| TEXAS INSTRUMENTS INCORPORATED
| Standard Linear and Logic Group
| IBIS Model of SN74LVC240A
| OCTAL BUFFER/DRIVER WITH 3-STATE OUTPUTS
| This file contains package information for the following:
|  SSOP 20-pin (DB) package as [Component] LVC240A_DB
|  TVSOP 20-pin (DGV) package as [Component] LVC240A_DGV
|  SOIC 20-pin (DW) package as [Component] LVC240A_DW
|  SOP 20-pin (NS) package as [Component] LVC240A_NS
|  TSSOP 20-pin (PW) package as [Component] LVC240A_PW
| This device can be powered at the following Vccs:
|  1.8 volt Vcc
|  2.5 volt Vcc
|  2.7 volt Vcc
|  3.3 volt Vcc
| This file provides unique models under the [Model Selector] for each Vcc.
| For operation at a specific Vcc, select the appropriate model after each
| [Model Selector] keyword.
[IBIS Ver]   3.2
[Comment char]  |_char
[File Name]   sn74lvc240a.ibs
[File Rev]   1.1 | e_die
[Date]   March 10, 2003
[Source]   Data created from TI-SPICE simulations at TI-SLL.
[Notes]   The following is an IBIS list for the LVC240A.
   Please contact sllibis@ti.com with questions and
   comments concerning SLL IBIS models.
   This IBIS model is created from a BA (back annotated
   netlist).
   - Power-clamp data has been deleted since there is no
   power-clamp diode in the device.
   - Due to the fact that the device is 5-V input
   tolerant, the pullup data has some non-monotonic warnings.
[Disclaimer] Property of Texas Instruments Incorporated.  Unauthorized
   reproduction and/or distribution is strictly prohibited.
   This product is protected under copyright law.
   Created  2003, (C) Copyright  2003, Texas Instruments
   Incorporated, All Rights Reserved
   UNLESS THERE IS A SIGNED, WRITTEN AGREEMENT TO THE
   CONTRARY, TEXAS INSTRUMENTS (TI) IS PROVIDING THE IBIS
   MODELS  AND WITHOUT ANY WARRANTY, EXPRESSED OR
   IMPLIED.  TI assumes no liability for:
   1) the accuracy of the IBIS models provided to your
   company;
   2) the proper functioning of these IBIS Models in your
   design or for any resulting applications; or
   3) infringement of patents, copyrights or intellectual
   property rights resulting from your use of these IBIS
   models.
   TI provides IBIS Models as a service to our customers.
   You and your company shall not distribute, sell or give
   these models to anyone else without prior written
   permission from TI.
   TI reserves the right to make changes to our products or
   to discontinue any semiconductor product or service
   without notice, and advises our customers to obtain the
   latest version of relevant information to verify, before
   placing orders, that the information being relied on is
   current.
   Please be aware that your receipt and use of the IBIS
   information provided shall serve as acceptance of these
   terms and conditions.  If you do not accept these terms,
   you should return or destroy the IBIS models and any
   other accompanying information immediately.
| Component LVC240A_DB 20-pin SSOP
[Component]   LVC240A_DB
[Manufacturer]   Texas Instruments, Inc.
[Package]
|   typ   min   max
R_pkg   4.000e-02   3.500e-02   5.100e-02
L_pkg   3.495e-09   3.035e-09   4.314e-09
C_pkg   4.200e-13   3.460e-13   5.020e-13
[Pin]   signal_name   model_name   R_pin   L_pin   C_pin
1   1NOE   LVC240A_OE   4.900e-02   4.310e-09   5.020e-13
2   1A1   LVC240A_IN   4.800e-02   3.903e-09   4.870e-13
3   2Y4   LVC240A_OUT   3.500e-02   3.189e-09   3.960e-13
4   1A2   LVC240A_IN   3.500e-02   3.036e-09   3.470e-13
5   2Y3   LVC240A_OUT   3.500e-02   3.035e-09   3.670e-13
6   1A3   LVC240A_IN   3.500e-02   3.035e-09   3.670e-13
7   2Y2   LVC240A_OUT   3.500e-02   3.036e-09   3.470e-13
8   1A4   LVC240A_IN   3.500e-02   3.189e-09   3.970e-13
9   2Y1   LVC240A_OUT   4.700e-02   3.899e-09   4.880e-13
10   GND   GND   5.100e-02   4.314e-09   5.000e-13
11   2A1   LVC240A_IN   5.100e-02   4.314e-09   5.000e-13
12   1Y4   LVC240A_OUT   4.700e-02   3.899e-09   4.880e-13
13   2A2   LVC240A_IN   3.500e-02   3.189e-09   3.970e-13
14   1Y3   LVC240A_OUT   3.500e-02   3.036e-09   3.460e-13
15   2A3   LVC240A_IN   3.500e-02   3.035e-09   3.670e-13
16   1Y2   LVC240A_OUT   3.500e-02   3.035e-09   3.670e-13
17   2A4   LVC240A_IN   3.500e-02   3.036e-09   3.460e-13
18   1Y1   LVC240A_OUT   3.500e-02   3.189e-09   3.970e-13
19   2NOE   LVC240A_OE   4.700e-02   3.899e-09   4.880e-13
20   VCC   POWER   5.100e-02   4.314e-09   5.020e-13
| Component LVC240A_DGV 20-pin TVSOP
[Component]   LVC240A_DGV
[Manufacturer]   Texas Instruments, Inc.
[Package]
|   typ   min   max
R_pkg   4.400e-02   3.800e-02   4.800e-02
L_pkg   2.561e-09   2.236e-09   2.961e-09
C_pkg   3.420e-13   2.640e-13   4.460e-13
[Pin]   signal_name   model_name   R_pin   L_pin   C_pin
1   1NOE   LVC240A_OE   4.400e-02   2.935e-09   4.170e-13
2   1A1   LVC240A_IN   4.200e-02   2.869e-09   4.460e-13
3   2Y4   LVC240A_OUT   4.300e-02   2.399e-09   3.160e-13
4   1A2   LVC240A_IN   4.400e-02   2.236e-09   2.650e-13
5   2Y3   LVC240A_OUT   4.600e-02   2.278e-09   2.640e-13
6   1A3   LVC240A_IN   4.500e-02   2.274e-09   2.640e-13
7   2Y2   LVC240A_OUT   4.400e-02   2.285e-09   2.690e-13
8   1A4   LVC240A_IN   4.300e-02   2.452e-09   3.200e-13
9   2Y1   LVC240A_OUT   4.400e-02   2.900e-09   4.460e-13
10   GND   GND   4.400e-02   2.961e-09   4.180e-13
11   2A1   LVC240A_IN   4.500e-02   2.954e-09   4.180e-13
12   1Y4   LVC240A_OUT   4.200e-02   2.847e-09   4.430e-13
13   2A2   LVC240A_IN   4.500e-02   2.453e-09   3.190e-13
14   1Y3   LVC240A_OUT   4.500e-02   2.297e-09   2.690e-13
15   2A3   LVC240A_IN   4.800e-02   2.334e-09   2.680e-13
16   1Y2   LVC240A_OUT   4.800e-02   2.335e-09   2.670e-13
17   2A4   LVC240A_IN   4.600e-02   2.299e-09   2.680e-13
18   1Y1   LVC240A_OUT   4.600e-02   2.457e-09   3.200e-13
19   2NOE   LVC240A_OE   4.300e-02   2.848e-09   4.410e-13
20   VCC   POWER   3.800e-02   2.812e-09   4.080e-13
| Component LVC240A_DW 20-pin SOIC
[Component]   LVC240A_DW
[Manufacturer]   Texas Instruments, Inc.
[Package]
|   typ   min   max
R_pkg   3.800e-02   3.300e-02   4.500e-02
L_pkg   5.012e-09   4.110e-09   6.349e-09
C_pkg   7.170e-13   5.300e-13   8.680e-13
[Pin]   signal_name   model_name   R_pin   L_pin   C_pin
1   1NOE   LVC240A_OE   4.200e-02   6.336e-09   8.650e-13
2   1A1   LVC240A_IN   4.300e-02   5.542e-09   8.670e-13
3   2Y4   LVC240A_OUT   3.400e-02   4.714e-09   7.320e-13
4   1A2   LVC240A_IN   3.400e-02   4.377e-09   5.910e-13
5   2Y3   LVC240A_OUT   3.600e-02   4.130e-09   5.330e-13
6   1A3   LVC240A_IN   3.500e-02   4.111e-09   5.300e-13
7   2Y2   LVC240A_OUT   3.400e-02   4.284e-09   5.830e-13
8   1A4   LVC240A_IN   3.400e-02   4.634e-09   7.260e-13
9   2Y1   LVC240A_OUT   4.000e-02   5.518e-09   8.650e-13
10   GND   GND   4.300e-02   6.349e-09   8.660e-13
11   2A1   LVC240A_IN   4.100e-02   6.281e-09   8.610e-13
12   1Y4   LVC240A_OUT   4.500e-02   5.561e-09   8.680e-13
13   2A2   LVC240A_IN   3.300e-02   4.778e-09   7.420e-13
14   1Y3   LVC240A_OUT   3.500e-02   4.414e-09   5.960e-13
15   2A3   LVC240A_IN   3.500e-02   4.110e-09   5.330e-13
16   1Y2   LVC240A_OUT   3.600e-02   4.130e-09   5.330e-13
17   2A4   LVC240A_IN   3.400e-02   4.377e-09   5.910e-13
18   1Y1   LVC240A_OUT   3.400e-02   4.714e-09   7.310e-13
19   2NOE   LVC240A_OE   4.300e-02   5.569e-09   8.680e-13
20   VCC   POWER   4.200e-02   6.308e-09   8.640e-13
| Component LVC240A_NS 20-pin SOP
[Component]   LVC240A_NS
[Manufacturer]   Texas Instruments, Inc.
[Package]
|   typ   min   max
R_pkg   4.400e-02   2.900e-02   5.800e-02
L_pkg   3.666e-09   2.317e-09   5.115e-09
C_pkg   5.480e-13   3.160e-13   7.250e-13
[Pin]   signal_name   model_name   R_pin   L_pin   C_pin
1   1NOE   LVC240A_OE   5.800e-02   5.115e-09   7.250e-13
2   1A1   LVC240A_IN   5.300e-02   4.591e-09   7.240e-13
3   2Y4   LVC240A_OUT   4.900e-02   3.754e-09   5.720e-13
4   1A2   LVC240A_IN   2.900e-02   2.549e-09   3.880e-13
5   2Y3   LVC240A_OUT   3.100e-02   2.317e-09   3.160e-13
6   1A3   LVC240A_IN   3.100e-02   2.317e-09   3.160e-13
7   2Y2   LVC240A_OUT   2.900e-02   2.556e-09   3.990e-13
8   1A4   LVC240A_IN   4.900e-02   3.754e-09   5.790e-13
9   2Y1   LVC240A_OUT   5.300e-02   4.591e-09   7.240e-13
10   GND   GND   5.800e-02   5.115e-09   7.250e-13
11   2A1   LVC240A_IN   5.800e-02   5.115e-09   7.250e-13
12   1Y4   LVC240A_OUT   5.300e-02   4.591e-09   7.240e-13
13   2A2   LVC240A_IN   4.900e-02   3.754e-09   5.790e-13
14   1Y3   LVC240A_OUT   2.900e-02   2.557e-09   3.990e-13
15   2A3   LVC240A_IN   3.100e-02   2.317e-09   3.160e-13
16   1Y2   LVC240A_OUT   3.100e-02   2.317e-09   3.160e-13
17   2A4   LVC240A_IN   2.900e-02   2.557e-09   3.990e-13
18   1Y1   LVC240A_OUT   4.900e-02   3.754e-09   5.790e-13
19   2NOE   LVC240A_OE   5.300e-02   4.591e-09   7.240e-13
20   VCC   POWER   5.800e-02   5.115e-09   7.250e-13
| Component LVC240A_PW 20-pin TSSOP
[Component]   LVC240A_PW
[Manufacturer]   Texas Instruments, Inc.
[Package]
|   typ   min   max
R_pkg   5.000e-02   4.200e-02   6.000e-02
L_pkg   2.802e-09   2.248e-09   3.553e-09
C_pkg   3.170e-13   2.020e-13   4.430e-13
[Pin]   signal_name   model_name   R_pin   L_pin   C_pin
1   1NOE   LVC240A_OE   5.500e-02   3.461e-09   4.400e-13
2   1A1   LVC240A_IN   5.500e-02   3.150e-09   4.010e-13
3   2Y4   LVC240A_OUT   4.200e-02   2.619e-09   3.020e-13
4   1A2   LVC240A_IN   4.500e-02   2.273e-09   2.020e-13
5   2Y3   LVC240A_OUT   4.500e-02   2.248e-09   2.240e-13
6   1A3   LVC240A_IN   4.500e-02   2.273e-09   2.260e-13
7   2Y2   LVC240A_OUT   4.400e-02   2.323e-09   2.050e-13
8   1A4   LVC240A_IN   4.600e-02   2.704e-09   3.070e-13
9   2Y1   LVC240A_OUT   6.000e-02   3.265e-09   4.110e-13
10   GND   GND   5.700e-02   3.506e-09   4.360e-13
11   2A1   LVC240A_IN   5.800e-02   3.553e-09   4.370e-13
12   1Y4   LVC240A_OUT   5.800e-02   3.193e-09   4.050e-13
13   2A2   LVC240A_IN   4.200e-02   2.704e-09   3.110e-13
14   1Y3   LVC240A_OUT   4.600e-02   2.392e-09   2.100e-13
15   2A3   LVC240A_IN   4.700e-02   2.334e-09   2.290e-13
16   1Y2   LVC240A_OUT   4.700e-02   2.300e-09   2.270e-13
17   2A4   LVC240A_IN   4.700e-02   2.349e-09   2.070e-13
18   1Y1   LVC240A_OUT   4.500e-02   2.677e-09   3.060e-13
19   2NOE   LVC240A_OE   6.000e-02   3.235e-09   4.060e-13
20   VCC   POWER   5.600e-02   3.487e-09   4.430e-13
| Model LVC240A_IN
[Model Selector]   LVC240A_IN
LVC240A_IN_18   1.8 volt Vcc
LVC240A_IN_25   2.5 volt Vcc
LVC240A_IN_33   3.3 volt Vcc
| Model LVC240A_OE
[Model Selector]   LVC240A_OE
LVC240A_OE_18   1.8 volt Vcc
LVC240A_OE_25   2.5 volt Vcc
LVC240A_OE_33   3.3 volt Vcc
| Model LVC240A_OUT
[Model Selector]   LVC240A_OUT
LVC240A_OUT_18   1.8 volt Vcc
LVC240A_OUT_25   2.5 volt Vcc
LVC240A_OUT_33   3.3 volt Vcc
| Models and submodels in the file (9): LVC240A_IN_18 (Input), LVC240A_IN_25 (Input), LVC240A_IN_33 (Input), LVC240A_OE_18 (Input), LVC240A_OE_25 (Input), LVC240A_OE_33 (Input), LVC240A_OUT_18 (3-state), LVC240A_OUT_25 (3-state), LVC240A_OUT_33 (3-state)
